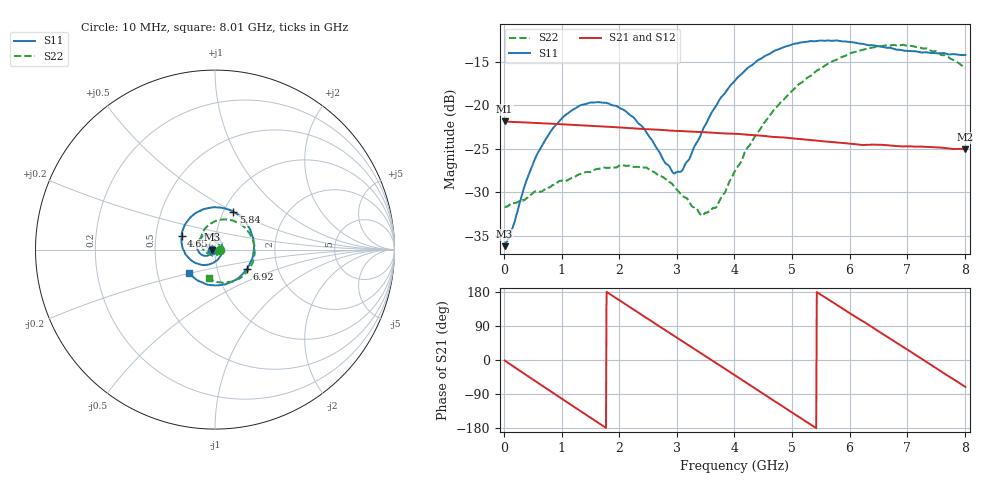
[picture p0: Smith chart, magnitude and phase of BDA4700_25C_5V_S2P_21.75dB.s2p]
!Agilent Technologies,E5071B,MY42404982,A.09.10
!Date: Mon Oct 20 13:37:19 2025
!Data & Calibration Information:
!Freq	S11:SOLT2(ON)	S21:SOLT2(ON)	S12:SOLT2(ON)	S22:SOLT2(ON)
# Hz S RI R 50
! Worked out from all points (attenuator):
!   801 points, 10 MHz to 8.01 GHz, reference 50 ohm
!   highest |S21| = -21.84 dB at 10 MHz (marker M1); lowest = -25.0 dB at 8.01 GHz (marker M2)
!   lowest |S11| = -36.2 dB at 10 MHz (marker M3), VSWR 1.03, Z = 48.5 - j0.122 ohm
!   |S11| at or under -10 dB: start of sweep to end of sweep
!   |S22| runs from -32.7 to -13.0 dB; largest |S21 - S12| = 0.00066
!   S11 on the Smith chart (normalised r, x): 10 MHz: 0.97, -0.00; 4.65 GHz: 0.68, +0.11; 5.84 GHz: 1.11, +0.50; 6.92 GHz: 1.39, -0.32; 8.01 GHz: 0.73, -0.20
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1e7  -0.0154 -0.00126  0.0809 -0.00176  0.0809 -0.00181  0.0261 -0.000817
1.2e8  -0.0164 -0.0084  0.0784 -0.0176  0.0784 -0.0176  0.0265 -0.00578
3.8e8  -0.0259 -0.0253  0.0619 -0.0503  0.0618 -0.0504  0.0213 -0.0196
6e8  -0.0419 -0.0343  0.0379 -0.0694  0.0378 -0.0695  0.0128 -0.0291
1e9  -0.0804 -0.0241  -0.016 -0.0762  -0.016 -0.0763  -0.0147 -0.0339
1.35e9  -0.1001 0.0107  -0.0562 -0.0523  -0.0563 -0.0524  -0.0364 -0.0178
2.08e9  -0.0445 0.083  -0.0644 0.0373  -0.0644 0.0373  -0.0295 0.0341
2.41e9  0.00344 0.0749  -0.0334 0.0651  -0.0335 0.0652  -0.00511 0.0436
2.68e9  0.0321 0.0445  -0.000751 0.0723  -0.000676 0.0723  0.0135 0.0372
2.93e9  0.0407 0.00523  0.0292 0.0653  0.0291 0.0652  0.0252 0.0241
3.06e9  0.038 -0.0167  0.0428 0.0569  0.0425 0.0571  0.0277 0.0141
3.44e9  -0.00525 -0.0711  0.0676 0.019  0.0676 0.019  0.0183 -0.0146
3.69e9  -0.0536 -0.0851  0.0685 -0.0107  0.0685 -0.0109  -9.85e-06 -0.0261
4.01e9  -0.1219 -0.0666  0.0522 -0.0445  0.0522 -0.0444  -0.0328 -0.0259
4.65e9  -0.186 0.0784  -0.0159 -0.0639  -0.0158 -0.0641  -0.0795 0.0438
5.35e9  -0.0538 0.2276  -0.0626 -0.00779  -0.0626 -0.00803  -0.0151 0.149
5.84e9  0.1028 0.2105  -0.0463 0.0397  -0.0462 0.0397  0.0948 0.1627
6.24e9  0.1952 0.1133  -0.0116 0.0581  -0.011 0.0582  0.1792 0.1075
6.68e9  0.2114 -0.0356  0.0309 0.0501  0.031 0.0501  0.2203 -0.00149
6.92e9  0.1763 -0.1092  0.0474 0.0336  0.0474 0.0334  0.2121 -0.0682
7.47e9  0.0153 -0.1994  0.0545 -0.0182  0.0545 -0.0183  0.1062 -0.1751
8.01e9  -0.1444 -0.1309  0.0181 -0.053  0.0183 -0.0531  -0.0318 -0.1608
